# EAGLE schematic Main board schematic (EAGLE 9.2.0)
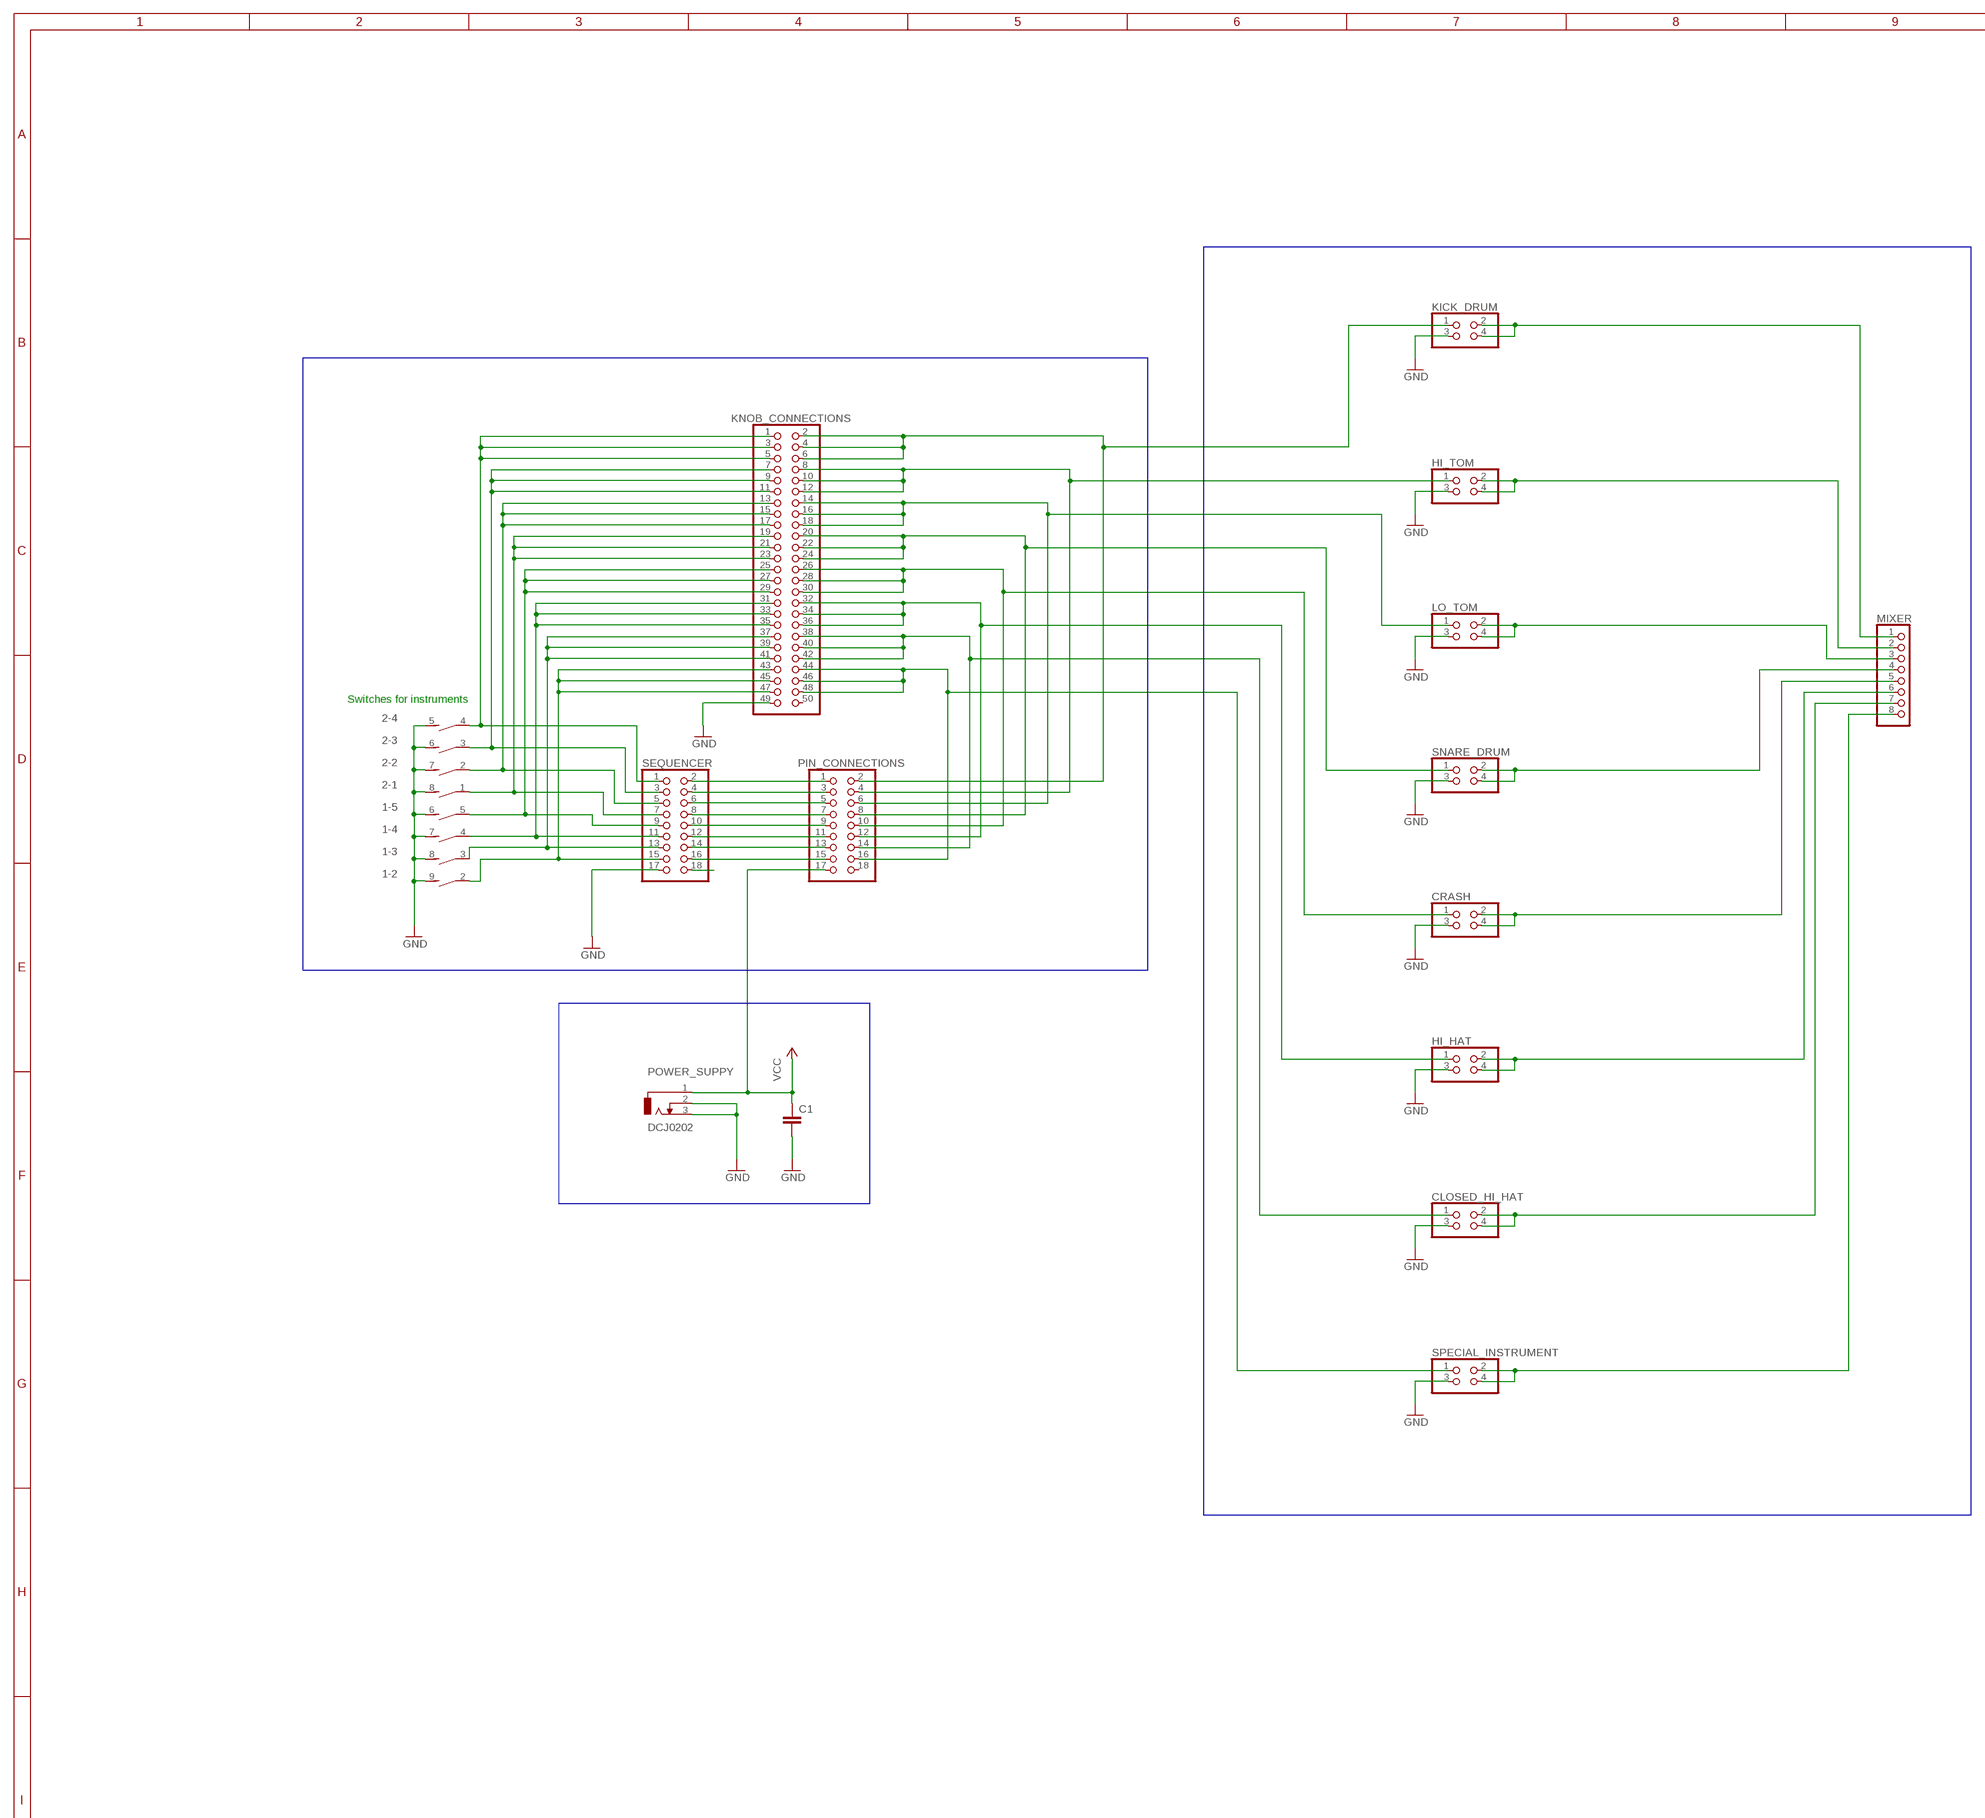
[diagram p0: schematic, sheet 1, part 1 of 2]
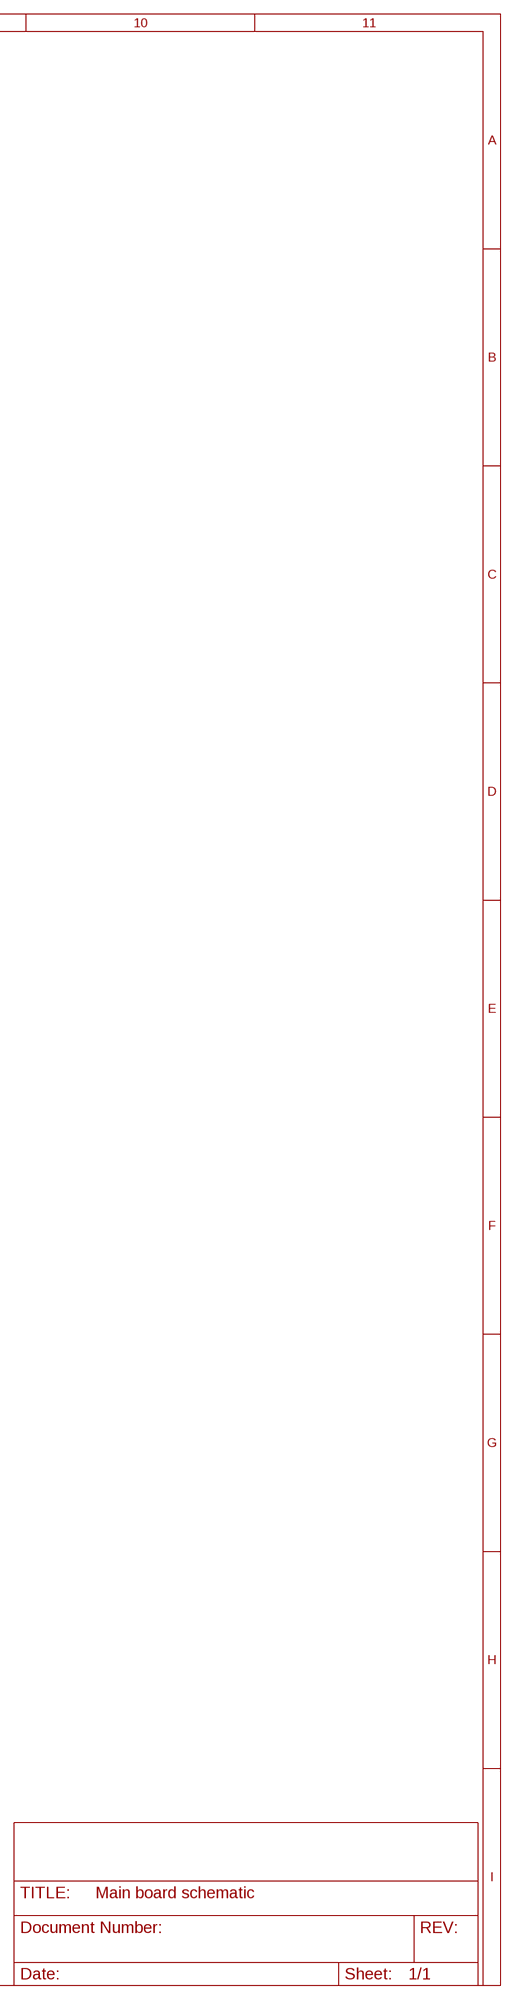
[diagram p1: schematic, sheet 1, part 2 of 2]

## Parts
1  DS05E  [DS-05]
2  DIP04S  [DIP04S]
C1  C2,5-3  [C2.5-3]
CLOSED_HI_HAT  PINHD-2X2  [2X02]
CRASH  PINHD-2X2  [2X02]
HI_HAT  PINHD-2X2  [2X02]
HI_TOM  PINHD-2X2  [2X02]
KICK_DRUM  PINHD-2X2  [2X02]
KNOB_CONNECTIONS  PINHD-2X25  [2X25]
LO_TOM  PINHD-2X2  [2X02]
MIXER  PINHD-1X8  [1X08]
PIN_CONNECTIONS  PINHD-2X9  [2X09]
POWER_SUPPY  DCJ0202  [DCJ0202]
SEQUENCER  PINHD-2X9  [2X09]
SNARE_DRUM  PINHD-2X2  [2X02]
SPECIAL_INSTRUMENT  PINHD-2X2  [2X02]

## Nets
GND: 1.6 1.7 1.8 1.9 2.5 2.6 2.7 2.8 C1.2 CLOSED_HI_HAT.3 CRASH.3 HI_HAT.3 HI_TOM.3 KICK_DRUM.3 KNOB_CONNECTIONS.49 LO_TOM.3 POWER_SUPPY.2 POWER_SUPPY.3 SEQUENCER.17 SNARE_DRUM.3 SPECIAL_INSTRUMENT.3
N$1: 2.3 KNOB_CONNECTIONS.7 KNOB_CONNECTIONS.9 KNOB_CONNECTIONS.11 SEQUENCER.3
N$2: 2.1 KNOB_CONNECTIONS.19 KNOB_CONNECTIONS.21 KNOB_CONNECTIONS.23 SEQUENCER.7
N$3: 1.5 KNOB_CONNECTIONS.25 KNOB_CONNECTIONS.27 KNOB_CONNECTIONS.29 SEQUENCER.9
N$4: 1.4 KNOB_CONNECTIONS.31 KNOB_CONNECTIONS.33 KNOB_CONNECTIONS.35 SEQUENCER.11
N$5: 1.3 KNOB_CONNECTIONS.37 KNOB_CONNECTIONS.39 KNOB_CONNECTIONS.41 SEQUENCER.13
N$6: KNOB_CONNECTIONS.14 KNOB_CONNECTIONS.16 KNOB_CONNECTIONS.18 LO_TOM.1 PIN_CONNECTIONS.6
N$8: 2.4 KNOB_CONNECTIONS.1 KNOB_CONNECTIONS.3 KNOB_CONNECTIONS.5 SEQUENCER.1
N$9: PIN_CONNECTIONS.1 SEQUENCER.2
N$10: 1.2 KNOB_CONNECTIONS.43 KNOB_CONNECTIONS.45 KNOB_CONNECTIONS.47 SEQUENCER.15
N$11: PIN_CONNECTIONS.3 SEQUENCER.4
N$12: PIN_CONNECTIONS.5 SEQUENCER.6
N$13: KNOB_CONNECTIONS.20 KNOB_CONNECTIONS.22 KNOB_CONNECTIONS.24 PIN_CONNECTIONS.8 SNARE_DRUM.1
N$14: HI_TOM.1 KNOB_CONNECTIONS.8 KNOB_CONNECTIONS.10 KNOB_CONNECTIONS.12 PIN_CONNECTIONS.4
N$15: PIN_CONNECTIONS.7 SEQUENCER.8
N$16: PIN_CONNECTIONS.9 SEQUENCER.10
N$17: PIN_CONNECTIONS.11 SEQUENCER.12
N$18: PIN_CONNECTIONS.13 SEQUENCER.14
N$19: PIN_CONNECTIONS.15 SEQUENCER.16
N$22: 2.2 KNOB_CONNECTIONS.13 KNOB_CONNECTIONS.15 KNOB_CONNECTIONS.17 SEQUENCER.5
N$23: CRASH.1 KNOB_CONNECTIONS.26 KNOB_CONNECTIONS.28 KNOB_CONNECTIONS.30 PIN_CONNECTIONS.10
N$24: HI_HAT.1 KNOB_CONNECTIONS.32 KNOB_CONNECTIONS.34 KNOB_CONNECTIONS.36 PIN_CONNECTIONS.12
N$25: KICK_DRUM.1 KNOB_CONNECTIONS.2 KNOB_CONNECTIONS.4 KNOB_CONNECTIONS.6 PIN_CONNECTIONS.2
N$26: KICK_DRUM.2 KICK_DRUM.4 MIXER.1
N$27: HI_TOM.2 HI_TOM.4 MIXER.2
N$28: CLOSED_HI_HAT.1 KNOB_CONNECTIONS.38 KNOB_CONNECTIONS.40 KNOB_CONNECTIONS.42 PIN_CONNECTIONS.14
N$29: KNOB_CONNECTIONS.44 KNOB_CONNECTIONS.46 KNOB_CONNECTIONS.48 PIN_CONNECTIONS.16 SPECIAL_INSTRUMENT.1
N$30: LO_TOM.2 LO_TOM.4 MIXER.3
N$32: MIXER.4 SNARE_DRUM.2 SNARE_DRUM.4
N$33: CRASH.2 CRASH.4 MIXER.5
N$34: HI_HAT.2 HI_HAT.4 MIXER.6
N$35: CLOSED_HI_HAT.2 CLOSED_HI_HAT.4 MIXER.7
N$36: MIXER.8 SPECIAL_INSTRUMENT.2 SPECIAL_INSTRUMENT.4
VCC: C1.1 PIN_CONNECTIONS.17 POWER_SUPPY.1
X: SEQUENCER.18
Unconnected: 1.1 1.10 KNOB_CONNECTIONS.50 PIN_CONNECTIONS.18

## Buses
B$1
B$2
B$3

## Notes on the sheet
- Switches for instruments

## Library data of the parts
1 = switch-dil:DS05E: DIL/CODE SWITCH; OC_FARNELL: unknown; OC_NEWARK: unknown
2 = switch-dil:DIP04S: DIL/CODE SWITCH; OC_FARNELL: unknown; OC_NEWARK: unknown
C1 = capacitor-wima:C: CAPACITOR
CLOSED_HI_HAT CRASH HI_HAT HI_TOM KICK_DRUM LO_TOM SNARE_DRUM SPECIAL_INSTRUMENT = pinhead:PINHD-2X2: PIN HEADER
KNOB_CONNECTIONS = pinhead:PINHD-2X25: PIN HEADER
MIXER = pinhead:PINHD-1X8: PIN HEADER
PIN_CONNECTIONS SEQUENCER = pinhead:PINHD-2X9: PIN HEADER
POWER_SUPPY = con-jack:DCJ0202: DC POWER JACK Source: DCJ0202.pdf; OC_FARNELL: unknown; OC_NEWARK: unknown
